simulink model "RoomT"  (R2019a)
settings: Solver=VariableStepAuto  StartTime=0.0  StopTime=tend  RelTol=1e-6
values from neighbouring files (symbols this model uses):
  ACmax = 4.5    [mainV3.m]    (also in mainV3_SRC.m)
  ACmin = 0    [mainV3.m]    (also in mainV3_SRC.m)
  EHmax = 4    [mainV3.m]    (also in mainV3_SRC.m)
  EHmin = 0    [mainV3.m]    (also in mainV3_SRC.m)
  HWmax = 3    [mainV3.m]    (also in mainV3_SRC.m)
  HWmin = 0    [mainV3.m]    (also in mainV3_SRC.m)
  Kc_ac = tau_ac/(K_ac*(tauc_ac+theta_ac))    (= -1.23666666667)    [RoomTuning.m]
  Kc_eh = tau_eh/(K_eh*(tauc_eh+theta_eh))    (= 1.23666666667)    [RoomTuning.m]
  Kc_hw = tau_hw/(K_hw*(tauc_hw+theta_hw))    (= 3.13641025641)    [RoomTuning.m]
  KI_ac = Kc_ac/tauI_ac    [RoomTuning.m]
  KI_eh = Kc_eh/tauI_eh    [RoomTuning.m]
  KI_hw = Kc_hw/tauI_hw    [RoomTuning.m]
  m_in0 = 0.4    [mainOL.m]    (also in mainV3.m; mainV3_SRC.m)
  p = [m,Cp, Ufl, Afl, mfl, Cpfl]'    [mainOL.m]    (also in mainV3.m; mainV3_SRC.m)
  par_ac = [p_ac, m_in0, Cp, kT]'    [mainV3.m]    (also in mainV3_SRC.m)
  par_el = [p_el, m_in0, Cp, kT]'    [mainV3.m]    (also in mainV3_SRC.m)
  par_hw = [p_hw, m_in0, Cp, kT]'    [mainV3.m]    (also in mainV3_SRC.m)
  par_J = [p_el, p_hw, p_ac, m_in0, kv, kT]'    [mainV3.m]    (also in mainV3_SRC.m)
  QAC0 = 0    [mainOL.m]    (also in mainV3.m; mainV3_SRC.m)
  QH10 = 0    [mainOL.m]    (also in mainV3.m; mainV3_SRC.m)
  QH20 = 0    [mainOL.m]    (also in mainV3.m; mainV3_SRC.m)
  Tback = 10    [mainV3.m]
  Tdes0 = T0    (= 21)    [mainV3.m]    (also in mainV3_SRC.m)
  Tin0 = 21    [mainOL.m]    (also in mainV3.m; mainV3_SRC.m)
  Tin_1 = 0    [mainOL.m]    (also in mainV3.m = 10; mainV3_SRC.m = 10)
  Tin_2 = 0    [mainOL.m]    (also in mainV3.m = -5; mainV3_SRC.m = -5)
  Tin_3 = -8    [mainV3.m]    (also in mainV3_SRC.m)
  Tin_4 = -13    [mainV3.m]    (also in mainV3_SRC.m)
  Tin_5 = +13    (= 13)    [mainV3.m]    (also in mainV3_SRC.m = 0)
  tTin_1 = 190000    [mainOL.m]    (also in mainV3.m = 1800; mainV3_SRC.m = 1800)
  tTin_2 = 2    [mainOL.m]    (also in mainV3.m = 12600; mainV3_SRC.m = 12600)
  tTin_3 = 7*3600    (= 25200)    [mainV3.m]    (also in mainV3_SRC.m)
  tTin_4 = 10*3600    (= 36000)    [mainV3.m]    (also in mainV3_SRC.m)
  tTin_5 = 10012.0*3600    (= 36043200)    [mainV3.m]    (also in mainV3_SRC.m = 20000)
  x0 = [T0; Tfl0]    [mainOL.m]    (also in mainV3.m; mainV3_SRC.m; col_obj.m = 0.5*ones(1,82)'; Simulate1Col.m = x)
undefined symbols (not defined in the file or in its folder): objRoom, Room, spQac, spQel, spQhw
libraries: simulink x3

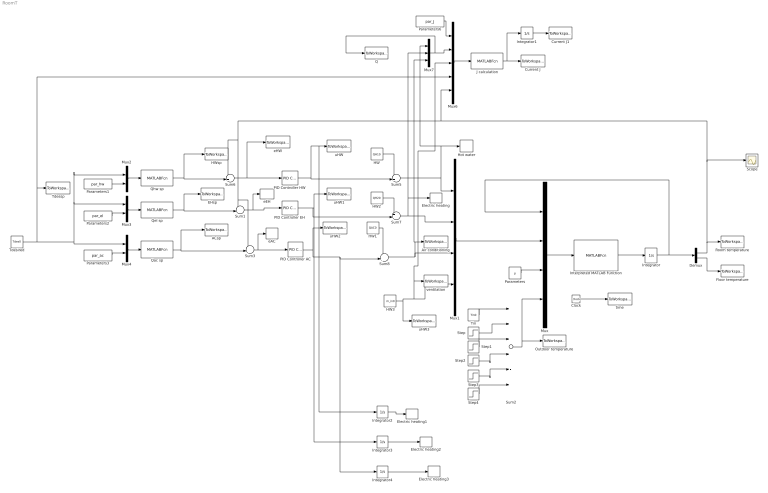
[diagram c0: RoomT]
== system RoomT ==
  ACsp : ToWorkspace  VariableName=ACsp  SampleTime=-1
  Air conditioning : ToWorkspace  VariableName=QAC  SampleTime=-1
  Clock : Clock
  Current J : ToWorkspace  VariableName=Jactual  SampleTime=-1
  Current J1 : ToWorkspace  VariableName=Jtot  SampleTime=-1
  Demux : Demux  Outputs=2
  EHsp : ToWorkspace  VariableName=EHsp  SampleTime=-1
  Electric heating : ToWorkspace  VariableName=QH2  SampleTime=-1
  Electric heating1 : ToWorkspace  VariableName=E_HW  SampleTime=-1
  Electric heating2 : ToWorkspace  VariableName=E_EH  SampleTime=-1
  Electric heating3 : ToWorkspace  VariableName=E_AC  SampleTime=-1
  Floor temperature : ToWorkspace  VariableName=Tfl  SampleTime=-1
  HW : Constant  Value=QH10
  HW1 : Constant  Value=QAC0
  HW2 : Constant  Value=QH20
  HW3 : Constant  Value=m_in0
  HWsp : ToWorkspace  VariableName=HWsp  SampleTime=-1
  Hot water : ToWorkspace  VariableName=QH1  SampleTime=-1
  Integrator : Integrator  InitialCondition=x0'
  Integrator{1..4} (4 alike) : Integrator
  Interpreted MATLAB Function : MATLABFcn  MATLABFcn=Room(u)  OutputDimensions=2  Output1D=off
  J calculation : MATLABFcn  MATLABFcn=objRoom(u)  OutputDimensions=1  Output1D=off
  Mux : Mux
  Mux1 : Mux
  Mux2 : Mux  Inputs=2
  Mux3 : Mux  Inputs=2
  Mux4 : Mux  Inputs=2
  Mux6 : Mux  Inputs=5
  Mux7 : Mux  Inputs=3
  Outdoor temperature : ToWorkspace  VariableName=Tin  SampleTime=-1
  PID Controller AC : simulink/Continuous/PID Controller  Controller=PI  Form=Parallel  TimeDomain=Continuous-time  SampleTime=-1  IntegratorMethod=Forward Euler  FilterMethod=Forward Euler  ControllerParametersSource=internal  P=Kc_ac  I=KI_ac  D=0  UseFilter=on  N=100  TunerSelectOption=Transfer Function Based (PID Tuner App)  ZeroCross=off  InitialConditionSource=internal  InitialConditionForIntegrator=0  InitialConditionForFilter=0  DifferentiatorICPrevScaledInput=0  ExternalReset=none  TrackingMode=off  Kt=1  LimitOutput=on  UpperSaturationLimit=ACmax  LowerSaturationLimit=ACmin  LinearizeAsGain=on  AntiWindupMode=back-calculation  Kb=1  POutMin=[]  POutMax=[]  IOutMin=[]  IOutMax=[]  DOutMin=[]  DOutMax=[]  NOutMin=[]  NOutMax=[]  SumOutMin=[]  SumOutMax=[]  SaturationOutMin=[]  SaturationOutMax=[]  PParamMin=[]  PParamMax=[]  IParamMin=[]  IParamMax=[]  DParamMin=[]  DParamMax=[]  NParamMin=[]  NParamMax=[]  KbParamMin=[]  KbParamMax=[]  KtParamMin=[]  KtParamMax=[]  KbOutMin=[]  KbOutMax=[]  KtOutMin=[]  KtOutMax=[]  IntegratorOutMin=[]  IntegratorOutMax=[]  FilterOutMin=[]  FilterOutMax=[]  SumI1OutMin=[]  SumI1OutMax=[]  SumI2OutMin=[]  SumI2OutMax=[]  SumI3OutMin=[]  SumI3OutMax=[]  SumI4OutMin=[]  SumI4OutMax=[]  SumDOutMin=[]  SumDOutMax=[]  DifferentiatorOutMin=[]  DifferentiatorOutMax=[]  FilterDiffOutCoefMin=[]  FilterDiffOutCoefMax=[]  ReciprocalOutMin=[]  ReciprocalOutMax=[]  SumDenOutMin=[]  SumDenOutMax=[]  SumNumOutMin=[]  SumNumOutMax=[]  DivideOutMin=[]  DivideOutMax=[]  IntegratorContinuousStateAttributes=''  IntegratorStateMustResolveToSignalObject=off  IntegratorRTWStateStorageClass=Auto  FilterContinuousStateAttributes=''  FilterStateMustResolveToSignalObject=off  FilterRTWStateStorageClass=Auto  ParallelPVariant=InternalParameters  IdealPVariant=Disabled  IVariant=InternalParameters  DVariant=Disabled  IntegratorVariant=Continuous  SatVariant=Enabled  AWVariant=BackCalculation  PCopyVariant=Disabled  TRVariant=Disabled  FdbkBlocksVariant=Forward  IdealPFdbkVariant=Disabled  SatFdbkVariant=Disabled  DerivativeFilterVariant=Disabled  NVariant=Disabled  NCopyVariant=Disabled_SignalSpec  FilterICVariant=Disabled  IntegratorICVariant=InternalICs  ExternalResetVariant=Disabled  TRSumVariant=Passthrough  SumFdbkVariant=Disabled  SumVariant=Sum_PI
  PID Controller EH : simulink/Continuous/PID Controller  Controller=PI  Form=Parallel  TimeDomain=Continuous-time  SampleTime=-1  IntegratorMethod=Forward Euler  FilterMethod=Forward Euler  ControllerParametersSource=internal  P=Kc_eh  I=KI_eh  D=0  UseFilter=on  N=100  TunerSelectOption=Transfer Function Based (PID Tuner App)  ZeroCross=off  InitialConditionSource=internal  InitialConditionForIntegrator=0  InitialConditionForFilter=0  DifferentiatorICPrevScaledInput=0  ExternalReset=none  TrackingMode=off  Kt=1  LimitOutput=on  UpperSaturationLimit=EHmax  LowerSaturationLimit=EHmin  LinearizeAsGain=on  AntiWindupMode=clamping  Kb=Tback  POutMin=[]  POutMax=[]  IOutMin=[]  IOutMax=[]  DOutMin=[]  DOutMax=[]  NOutMin=[]  NOutMax=[]  SumOutMin=[]  SumOutMax=[]  SaturationOutMin=[]  SaturationOutMax=[]  PParamMin=[]  PParamMax=[]  IParamMin=[]  IParamMax=[]  DParamMin=[]  DParamMax=[]  NParamMin=[]  NParamMax=[]  KbParamMin=[]  KbParamMax=[]  KtParamMin=[]  KtParamMax=[]  KbOutMin=[]  KbOutMax=[]  KtOutMin=[]  KtOutMax=[]  IntegratorOutMin=[]  IntegratorOutMax=[]  FilterOutMin=[]  FilterOutMax=[]  SumI1OutMin=[]  SumI1OutMax=[]  SumI2OutMin=[]  SumI2OutMax=[]  SumI3OutMin=[]  SumI3OutMax=[]  SumI4OutMin=[]  SumI4OutMax=[]  SumDOutMin=[]  SumDOutMax=[]  DifferentiatorOutMin=[]  DifferentiatorOutMax=[]  FilterDiffOutCoefMin=[]  FilterDiffOutCoefMax=[]  ReciprocalOutMin=[]  ReciprocalOutMax=[]  SumDenOutMin=[]  SumDenOutMax=[]  SumNumOutMin=[]  SumNumOutMax=[]  DivideOutMin=[]  DivideOutMax=[]  IntegratorContinuousStateAttributes=''  IntegratorStateMustResolveToSignalObject=off  IntegratorRTWStateStorageClass=Auto  FilterContinuousStateAttributes=''  FilterStateMustResolveToSignalObject=off  FilterRTWStateStorageClass=Auto  ParallelPVariant=InternalParameters  IdealPVariant=Disabled  IVariant=InternalParameters  DVariant=Disabled  IntegratorVariant=Continuous  SatVariant=Enabled  AWVariant=ContClampingParallel  PCopyVariant=Disabled  TRVariant=Disabled  FdbkBlocksVariant=Forward  IdealPFdbkVariant=Disabled  SatFdbkVariant=Disabled  DerivativeFilterVariant=Disabled  NVariant=Disabled  NCopyVariant=Disabled_SignalSpec  FilterICVariant=Disabled  IntegratorICVariant=InternalICs  ExternalResetVariant=Disabled  TRSumVariant=Passthrough  SumFdbkVariant=Disabled  SumVariant=Sum_PI
  PID Controller HW : simulink/Continuous/PID Controller  Controller=PI  Form=Parallel  TimeDomain=Continuous-time  SampleTime=-1  IntegratorMethod=Forward Euler  FilterMethod=Forward Euler  ControllerParametersSource=internal  P=Kc_hw  I=KI_hw  D=0  UseFilter=on  N=100  TunerSelectOption=Transfer Function Based (PID Tuner App)  ZeroCross=off  InitialConditionSource=internal  InitialConditionForIntegrator=0  InitialConditionForFilter=0  DifferentiatorICPrevScaledInput=0  ExternalReset=none  TrackingMode=off  Kt=1  LimitOutput=on  UpperSaturationLimit=HWmax  LowerSaturationLimit=HWmin  LinearizeAsGain=on  AntiWindupMode=clamping  Kb=Tback  POutMin=[]  POutMax=[]  IOutMin=[]  IOutMax=[]  DOutMin=[]  DOutMax=[]  NOutMin=[]  NOutMax=[]  SumOutMin=[]  SumOutMax=[]  SaturationOutMin=[]  SaturationOutMax=[]  PParamMin=[]  PParamMax=[]  IParamMin=[]  IParamMax=[]  DParamMin=[]  DParamMax=[]  NParamMin=[]  NParamMax=[]  KbParamMin=[]  KbParamMax=[]  KtParamMin=[]  KtParamMax=[]  KbOutMin=[]  KbOutMax=[]  KtOutMin=[]  KtOutMax=[]  IntegratorOutMin=[]  IntegratorOutMax=[]  FilterOutMin=[]  FilterOutMax=[]  SumI1OutMin=[]  SumI1OutMax=[]  SumI2OutMin=[]  SumI2OutMax=[]  SumI3OutMin=[]  SumI3OutMax=[]  SumI4OutMin=[]  SumI4OutMax=[]  SumDOutMin=[]  SumDOutMax=[]  DifferentiatorOutMin=[]  DifferentiatorOutMax=[]  FilterDiffOutCoefMin=[]  FilterDiffOutCoefMax=[]  ReciprocalOutMin=[]  ReciprocalOutMax=[]  SumDenOutMin=[]  SumDenOutMax=[]  SumNumOutMin=[]  SumNumOutMax=[]  DivideOutMin=[]  DivideOutMax=[]  IntegratorContinuousStateAttributes=''  IntegratorStateMustResolveToSignalObject=off  IntegratorRTWStateStorageClass=Auto  FilterContinuousStateAttributes=''  FilterStateMustResolveToSignalObject=off  FilterRTWStateStorageClass=Auto  ParallelPVariant=InternalParameters  IdealPVariant=Disabled  IVariant=InternalParameters  DVariant=Disabled  IntegratorVariant=Continuous  SatVariant=Enabled  AWVariant=ContClampingParallel  PCopyVariant=Disabled  TRVariant=Disabled  FdbkBlocksVariant=Forward  IdealPFdbkVariant=Disabled  SatFdbkVariant=Disabled  DerivativeFilterVariant=Disabled  NVariant=Disabled  NCopyVariant=Disabled_SignalSpec  FilterICVariant=Disabled  IntegratorICVariant=InternalICs  ExternalResetVariant=Disabled  TRSumVariant=Passthrough  SumFdbkVariant=Disabled  SumVariant=Sum_PI
  Parameters : Constant  Value=p
  Parameters1 : Constant  Value=par_hw
  Parameters2 : Constant  Value=par_el
  Parameters3 : Constant  Value=par_ac
  Parameters6 : Constant  Value=par_J
  Q : ToWorkspace  VariableName=Q  SampleTime=-1
  Qac sp : MATLABFcn  MATLABFcn=spQac(u)  OutputDimensions=1  Output1D=off
  Qel sp : MATLABFcn  MATLABFcn=spQel(u)  OutputDimensions=1  Output1D=off
  Qhw sp : MATLABFcn  MATLABFcn=spQhw(u)  OutputDimensions=1  Output1D=off
  Room temperature : ToWorkspace  VariableName=T  SampleTime=-1
  Scope : Scope
  Step : Step  Time=tTin_1  After=Tin_1  SampleTime=0
  Step1 : Step  Time=tTin_2  After=Tin_2  SampleTime=0
  Step2 : Step  Time=tTin_3  After=Tin_3  SampleTime=0
  Step3 : Step  Time=tTin_4  After=Tin_4  SampleTime=0
  Step4 : Step  Time=tTin_5  After=Tin_5  SampleTime=0
  Sum1 : Sum  Inputs=-+|
  Sum2 : Sum  Inputs=|++++++
  Sum3 : Sum  Inputs=-+|
  Sum5 : Sum  Inputs=++|
  Sum6 : Sum  Inputs=-+|
  Sum7 : Sum  Inputs=++|
  Sum8 : Sum  Inputs=++|
  Tdesired : Constant  Value=Tdes0
  Tdessp : ToWorkspace  VariableName=Tdes_sp  SampleTime=-1
  Tin : Constant  Value=Tin0
  eAC : ToWorkspace  VariableName=eAC  SampleTime=-1
  eEH : ToWorkspace  VariableName=eEH  SampleTime=-1
  eHW : ToWorkspace  VariableName=eHW  SampleTime=-1
  time : ToWorkspace  VariableName=t  SampleTime=-1
  uHW : ToWorkspace  VariableName=uHW  SampleTime=-1
  uHW1 : ToWorkspace  VariableName=uEH  SampleTime=-1
  uHW2 : ToWorkspace  VariableName=uAC  SampleTime=-1
  uHW3 : ToWorkspace  VariableName=u_mv  SampleTime=-1
  ventilation : ToWorkspace  VariableName=m_in  SampleTime=-1
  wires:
  Clock/1 -> time/1
  Interpreted MATLAB Function/1 -> Integrator/1
  Mux/1 -> Interpreted MATLAB Function/1
  Integrator/1 -> Demux/1, Mux/1
  Parameters/1 -> Mux/3
  Sum2/1 -> Mux/4, Outdoor temperature/1
  Step1/1 -> Sum2/3
  Step/1 -> Sum2/2
  Tin/1 -> Sum2/1
  Mux1/1 -> Mux/2
  Demux/1 -> Mux6/5, Sum6/1, Sum3/1, Sum1/1, Scope/1, Room temperature/1
  Demux/2 -> Floor temperature/1
  Tdesired/1 -> Mux6/4, Tdessp/1, Mux3/1, Mux2/1, Mux4/1
  Qhw sp/1 -> Sum6/2, HWsp/1
  Mux2/1 -> Qhw sp/1
  Mux3/1 -> Qel sp/1
  Mux4/1 -> Qac sp/1
  Parameters1/1 -> Mux2/2
  Parameters2/1 -> Mux3/2
  Parameters3/1 -> Mux4/2
  Qel sp/1 -> EHsp/1, Sum1/2
  Qac sp/1 -> ACsp/1, Sum3/2
  Sum3/1 -> eAC/1, PID Controller AC/1
  Sum6/1 -> eHW/1, PID Controller HW/1
  PID Controller HW/1 -> Integrator2/1, uHW/1, Sum5/2
  Sum1/1 -> eEH/1, PID Controller EH/1
  PID Controller EH/1 -> Integrator3/1, uHW1/1, Sum7/2
  PID Controller AC/1 -> uHW2/1, Integrator4/1, Sum8/2
  Sum5/1 -> Mux1/1, Mux7/1, Hot water/1
  HW/1 -> Sum5/1
  Sum7/1 -> Mux7/2, Electric heating/1, Mux1/2
  HW2/1 -> Sum7/1
  Sum8/1 -> Mux7/3, Air conditioning/1, Mux1/3
  HW1/1 -> Sum8/1
  Step2/1 -> Sum2/4
  Step3/1 -> Sum2/5
  Step4/1 -> Sum2/6
  J calculation/1 -> Integrator1/1, Current J/1
  Mux6/1 -> J calculation/1
  HW3/1 -> Mux6/3, ventilation/1, Mux1/4, uHW3/1
  Parameters6/1 -> Mux6/1
  Mux7/1 -> Q/1, Mux6/2
  Integrator1/1 -> Current J1/1
  Integrator2/1 -> Electric heating1/1
  Integrator3/1 -> Electric heating2/1
  Integrator4/1 -> Electric heating3/1
